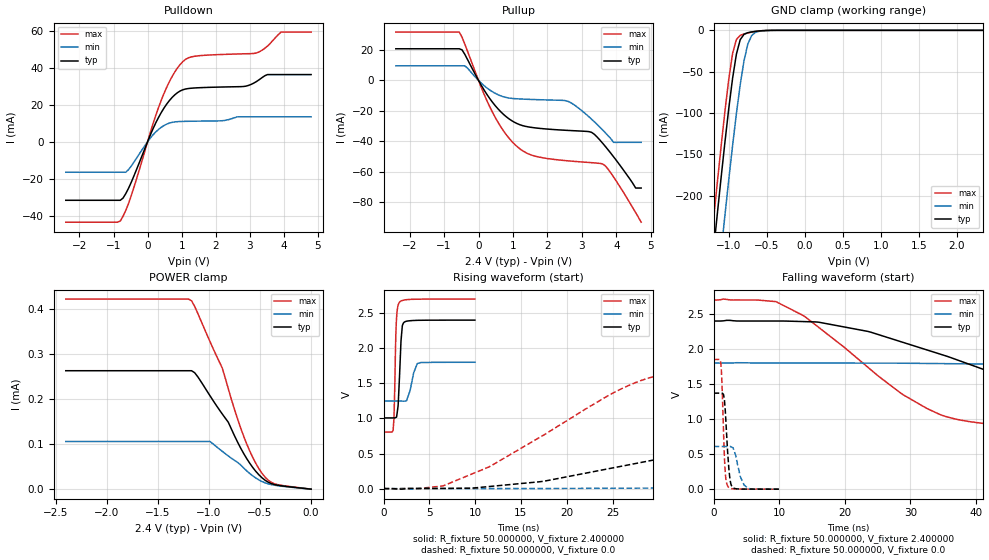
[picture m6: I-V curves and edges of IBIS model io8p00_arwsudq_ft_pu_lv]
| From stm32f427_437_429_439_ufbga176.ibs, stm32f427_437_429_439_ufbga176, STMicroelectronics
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|   Model io8p00_arwsudq_ft_pu_lv
[Model]  io8p00_arwsudq_ft_pu_lv
Model_type I/O
Polarity   Non-Inverting
Enable   Active-Low
Vinl =   0.720000V
Vinh =   1.680000V
Vmeas =  1.200000V
Cref =   50.000000pF
Rref =   100.000000M
Vref =   0.0V
C_comp   2.828000pF   2.774600pF   2.917100pF
[Temperature Range]   25.000000   0.125000k   -40.000000
[Pullup Reference]   2.400000V   1.800000V   2.700000V
[Pulldown Reference]   0.0V   0.0V   0.0V
[POWER Clamp Reference]   2.400000V   1.800000V   2.700000V
[GND Clamp Reference]   0.0V   0.0V   0.0V
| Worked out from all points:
|   slope of the pulldown table from 0 to 0.36 V, typ, clamps not added: 25 ohm
|   slope of the pullup table from 0 to 0.36 V, typ, clamps not added: 27.7 ohm
|   GND clamp passes 1 mA (typ) near -0.62 V on its own axis
|   rising waveform, R_fixture 50.000000, V_fixture 2.400000: 20-80 % time 288ps typ, 616ps min, 205ps max; typ from 1.01 V to 2.4 V
|   rising waveform, R_fixture 50.000000, V_fixture 0.0: 20-80 % time 30.9ns typ, 81ns min, 14.7ns max; typ from 0.001 V to 1.37 V
|   falling waveform, R_fixture 50.000000, V_fixture 2.400000: 20-80 % time 29.6ns typ, 76ns min, 16.1ns max; typ from 2.4 V to 1.01 V
|   falling waveform, R_fixture 50.000000, V_fixture 0.0: 20-80 % time 541ps typ, 1ns min, 412ps max; typ from 1.37 V to 0.001 V
[Pulldown]
|Voltage   I(typ)   I(min)   I(max)
-2.4V     -31.67mA   -16.51mA   -43.52mA
-800mV    -31.67mA   -16.51mA   -42.87mA
-480mV    -21.98mA   -13.17mA   -29.21mA
80mV      3.63mA     1.966mA    5.012mA
480mV     18.16mA    8.738mA    26.02mA
800mV     25.38mA    10.72mA    37.77mA
1.12V     28.53mA    11.02mA    44.6mA
2.8V      29.84mA    13.46mA    47.53mA
3.2V      32.6mA     13.46mA    48.03mA
3.52V     36.31mA    13.46mA    51.75mA
3.92V     36.31mA    13.46mA    59.29mA
4.8V      36.31mA    13.46mA    59.29mA
[Pullup]
|Voltage   I(typ)   I(min)   I(max)
-2.4V     20.87mA    9.66mA     31.87mA
-560mV    20.87mA    9.66mA     31.87mA
-400mV    17.27mA    9.66mA     24.06mA
320mV     -11.75mA   -6.207mA   -17.08mA
960mV     -26.47mA   -11.82mA   -40.02mA
1.52V     -30.88mA   -12.51mA   -49.05mA
2.56V     -32.88mA   -13.48mA   -52.9mA
3.28V     -34.19mA   -25.52mA   -54.17mA
3.6V      -41.32mA   -32.62mA   -54.98mA
3.92V     -50.34mA   -40.8mA    -63.65mA
4.56V     -70.9mA    -40.8mA    -87.11mA
4.72V     -70.9mA    -40.8mA    -93.4mA
[GND_clamp]
|Voltage   I(typ)   I(min)   I(max)
-2.4V     -1.425A    -1.509A    -1.395A
-1.25V    -311.8mA   -402mA     -274.5mA
-1.2V     -266mA     -356.2mA   -228.4mA
-1.15V    -220.9mA   -310.9mA   -183.1mA
-1.1V     -176.9mA   -266.3mA   -139mA
-1.05V    -134.3mA   -222.6mA   -97.01mA
-950mV    -57.81mA   -139.1mA   -27.86mA
-900mV    -28.73mA   -100.5mA   -11.04mA
-850mV    -11.29mA   -65.69mA   -6.054mA
-750mV    -2.852mA   -16.6mA    -3.179mA
-600mV    -750uA     -1.167mA   -738.5uA
2.35V     0A         0A         0A
[POWER_clamp]
|Voltage   I(typ)   I(min)   I(max)
-2.4V     263.2uA    106uA      422.4uA
-1.17V    263.2uA    106uA      418.5uA
-1.11V    250.1uA    106uA      391.1uA
-990mV    207.7uA    106uA      328.2uA
-870mV    167.2uA    84.17uA    269.6uA
-810mV    148.5uA    73.71uA    222.7uA
-660mV    79.21uA    47.09uA    117.6uA
-570mV    47.82uA    29.3uA     69.9uA
-510mV    31.66uA    20.4uA     45.18uA
-420mV    15.55uA    11.87uA    19.89uA
-360mV    10.34uA    8.845uA    12.09uA
0V        0A         0A         0A
[Ramp]
| variable   typ   min   max
dV/dt_r  0.82315/30.92269n   0.36270/83.29207n   1.11082/14.64109n
dV/dt_f  0.83592/29.60361n   0.32640/76.33889n   1.13649/16.04783n
R_load = 50.000000
[Rising Waveform]
R_fixture= 50.000000
V_fixture= 2.400000
V_fixture_min= 1.800000
V_fixture_max= 2.700000
|time   V(typ)   V(min)   V(max)
0s        1.007V     1.247V     805.7mV
1.041ns   1.007V     1.247V     832.1mV
1.141ns   1.007V     1.247V     1.03V
1.381ns   1.017V     1.247V     2.339V
1.582ns   1.174V     1.247V     2.608V
1.722ns   1.543V     1.247V     2.652V
1.902ns   2.099V     1.247V     2.672V
2.262ns   2.371V     1.246V     2.686V
3.684ns   2.397V     1.781V     2.698V
9.97ns    2.4V       1.8V       2.7V
[Rising Waveform]
R_fixture= 50.000000
V_fixture= 0.0
V_fixture_min= 0.0
V_fixture_max= 0.0
|time   V(typ)   V(min)   V(max)
0s        881.8uV    840.3uV    927.4uV
6.507ns   3.56mV     1.878mV    40mV
11.51ns   30.16mV    1.904mV    309.7mV
24.52ns   282.7mV    5.594mV    1.325V
28.53ns   383.7mV    7.728mV    1.558V
43.54ns   826.5mV    45.48mV    1.797V
60.06ns   1.175V     97.1mV     1.84V
80.58ns   1.318V     198.3mV    1.848V
148.1ns   1.369V     495.1mV    1.852V
249.2ns   1.371V     610.3mV    1.852V
[Falling Waveform]
R_fixture= 50.000000
V_fixture= 2.400000
V_fixture_min= 1.800000
V_fixture_max= 2.700000
|time   V(typ)   V(min)   V(max)
0s        2.4V       1.8V       2.7V
9.51ns    2.4V       1.8V       2.677V
14.01ns   2.391V     1.8V       2.456V
23.52ns   2.252V     1.799V     1.741V
32.53ns   1.987V     1.795V     1.152V
46.55ns   1.537V     1.771V     894.7mV
62.06ns   1.22V      1.713V     845mV
89.59ns   1.069V     1.55V      817.2mV
145.1ns   1.016V     1.347V     806.8mV
249.2ns   1.007V     1.247V     805.7mV
[Falling Waveform]
R_fixture= 50.000000
V_fixture= 0.0
V_fixture_min= 0.0
V_fixture_max= 0.0
|time   V(typ)   V(min)   V(max)
0s        1.371V     610.3mV    1.852V
1.061ns   1.371V     610.2mV    1.822V
1.261ns   1.371V     610.2mV    1.541V
1.682ns   1.241V     610mV      391.3mV
1.862ns   990mV      609.7mV    154.5mV
2.142ns   528.4mV    609.9mV    46.47mV
2.503ns   138.4mV    612.2mV    14.29mV
2.983ns   20.64mV    586.9mV    5.519mV
4.645ns   2.122mV    61.64mV    1.988mV
9.97ns    881.8uV    840.3uV    927.4uV
